(* Logix 5000 AddOnInstructionDefinition export AMP_Point_to_Point_IO; software revision 20.04 *)

TYPE AMP_Status_Word :   // Applied Motion Input Assembly Status Word
STRUCT
   Enabled : BOOL;   // Motor Enabled (Motor Disabled if this bit = 0)
   Sampling : BOOL;   // Sampling (for Quick Tuner)
   Drive_Fault : BOOL;   // Drive Fault (check Alarm Code)
   In_Position : BOOL;   // In Position (motor is in position)
   Moving : BOOL;   // Moving (motor is moving)
   Jogging : BOOL;   // Jogging (currently in jog mode)
   Stopping : BOOL;   // Stopping (in the process of stopping from a stop command)
   Waiting : BOOL;   // Waiting (for an input; executing a WI command)
   Saving : BOOL;   // Saving (parameter data is being saved)
   Alarm_Present : BOOL;   // Alarm present (check Alarm Code)
   Homing : BOOL;   // Homing (executing an SH command)
   Wait_Time : BOOL;   // Waiting (for time; executing a WD or WT command)
   Wizard_Running : BOOL;   // Wizard running (Timing Wizard is running)
   Checking_Encoder : BOOL;   // Checking encoder (Timing Wizard is running)
   Q_Program_Running : BOOL;   // Q Program is running
   Initializing : BOOL;   // Initializing (happens at power up) ; Servo Ready (for SV200 drives only)
END_STRUCT
END_TYPE

TYPE AMP_Input_Assembly_v2 :   // Applied Motion Drive Input Assembly Version 2.0
STRUCT
   Status_Code : DINT;   // Status Code
   Alarm_Code : DINT;   // Alarm Code
   Voltage : DINT;   // Supply Voltage (x0.1V)
   Current : DINT;   // Actual Current (mA)
   Temp : DINT;   // Drive Temperature (0.1 deg C)
   Encoder_Position : DINT;   // Encoder Position (20,000 counts = 1 shaft turn)
   Absolute_Position : DINT;   // Absolute Position (20,000 counts = 1 shaft turn)
   Position_Error : DINT;   // Position Error (counts)
   Actual_Velocity : DINT;   // Actual Velocity (rev/sec * 240, 0 when no encoder)
   Extended_Inputs : DINT;   // Input Status (Extended)
   Main_Board_Inputs : DINT;   // Input Status (Main board)
   Word11 : DINT;   // Reserved
   Analog_Input_1 : DINT;   // Analog Input 1 (ADC counts, 0=min V, 16383 = max V)
   Analog_Input_2 : DINT;   // Analog Input 2 (ADC counts, 0=min V, 16383 = max V)
END_STRUCT
END_TYPE

ADD_ON_INSTRUCTION AMP_Point_to_Point_IO   (* revision 1.0 *)
// Applied Motion - Point to Point Move with IO AOI
// Help:
// The Point-to-Point Move with I/O AOI executes moves involving up to 2 Input conditions and a possible output state change. The move variant can be any of the following:
// - FS - Feed to Sensor
// - FD - Feed to Double Sensor
// - FM - Feed to Sensor with Mask Distance
// - FY - Feed to Sensor with Safety Distance
// - FO - Feed to Length and Set Output
// - FE - Follow Encoder
// - SH - Seek Home
// All seven (7) of the above variants need exactly one I/O point except for FD which requires a second I/O point to be specified in the parameters.
VAR_IN_OUT
   Input : DINT[14]; {required}   // Drive Input Assembly
   Output : DINT[16]; {required}   // Drive Output Assembly
        [0]   // Command Word
        [1]   // Jog Speed (0.25 rev/min)
        [2]   // Jog Acceleration (10 rev/s/s)
        [3]   // Jog Deceleration (10 rev/s/s)
        [4]   // Point-to-Point Velocity (0.25 rev/min)
        [5]   // Point-to-Point Acceleration (10 rev/s/s)
        [6]   // Point-to-Point Deceleration (10 rev/s/s)
        [7]   // Point-to-Point Distance (Motor steps)
        [9]   // (2x ASCII Letters in 16 lower word)
        [10]   // Data/Register 1
        [11]   // Data/Register 2
END_VAR
VAR_INPUT
   RPI : DINT := 100; {visible}   // Drive Connection Request Packet Interval (milliseconds)
   Start : BOOL; {required}   // Start the Move
   Command : INT := 'FE'; {required}   // Command variant: FS/FD/FY/FM/FO/SH/FE
   IO1_Number : DINT; {required}   // Main Input/Output Number (0 = Encoder index, 1-8 = In/Out 1-8)
   IO1_Condition : SINT := 'R'; {required}   // Main Input/Output Condition/State H/L/R/F (High/Low/Rising Edge/Falling Edge)
   IO2_Number : DINT; {required}   // Second Input/Output Number (0 = Encoder index, 1-8 = In/Out 1-8)
   IO2_Condition : SINT; {required}   // Second Input/Output Condition/State H/L/R/F (High/Low/Rising Edge/Falling Edge)
   IO_Connector : DINT := 1; {required}   // I/O Connector (1=IN/OUT 1, 2=IN/OUT 2)
   Distance : DINT; {required}   // Distance to Move (negative = reverse)
   Speed : REAL; {required}   // Velocity of Move (rev/min)
   Acc : REAL; {required}   // Acceleration of Move (rev/s/s)
   Dec : REAL; {required}   // Deceleration (rev/s/s)
   Change_Distance : DINT; {required}   // Change Distance (steps, FY/FM/FO only)
   Change_Speed : REAL; {required}   // Velocity Change (rev/s) (FD only)
END_VAR
VAR_OUTPUT
   Sent : BOOL; {access Read Only, visible}   // Move has been sent to drive
   In_Progress : BOOL; {access Read Only, visible}   // Move in progress
   Done : BOOL; {access Read Only, visible}   // Move completed without errors - desired position reached
   Error : BOOL; {access Read Only, visible}   // Move failed to complete - drive not ready or faulted
   State : DINT := 10; {access Read Only}   // Internal state of progress
END_VAR
VAR
   Loc_StatusCode : AMP_Status_Word;
   Loc_CommandOff_Timer : TIMER;   // Timer to make sure command value was 0 before sending a new command
   Loc_CommandOn_Timer : TIMER;   // Timer to make sure command value is set long enough to be sent to drive
   Loc_Input_Assembly : AMP_Input_Assembly_v2; {access None}
   Loc_Start_ONS : BOOL; {access None}
   Loc_ChangeSpeed_Required : BOOL; {access None}
   Loc_ChangeDistance_Required : BOOL; {access None}
   Loc_IO1_Condition_Encoded : INT; {access None}
   Loc_IO1_Number_Encoded : INT; {access None}
   Loc_IO2_Condition_Encoded : INT; {access None}
   Loc_IO2_Number_Encoded : INT; {access None}
END_VAR

ROUTINE Logic   (* ladder *)
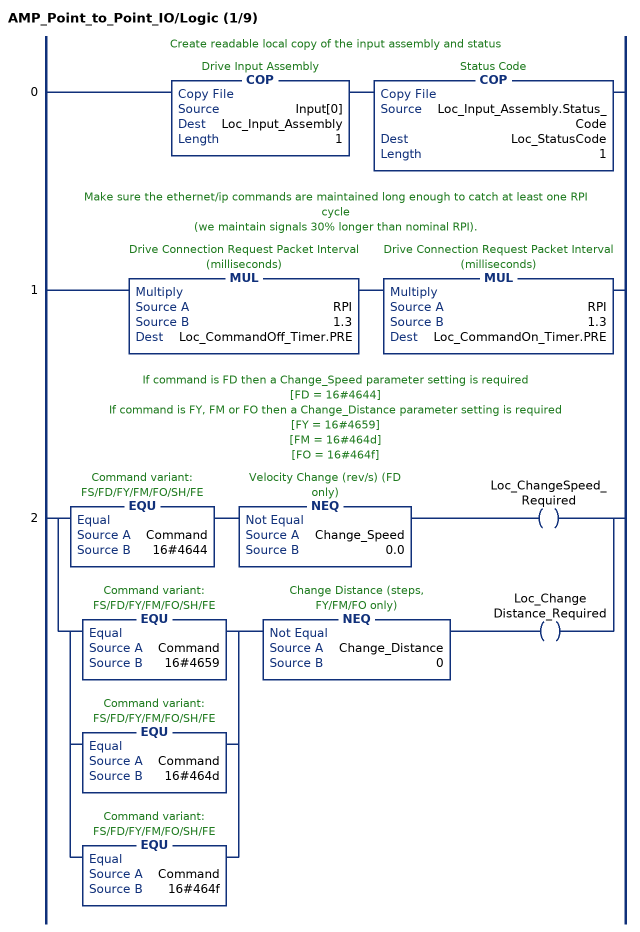
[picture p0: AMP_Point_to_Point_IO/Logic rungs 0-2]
   // Create readable local copy of the input assembly and status
   0: COP(Input[0],Loc_Input_Assembly,1)COP(Loc_Input_Assembly.Status_Code,Loc_StatusCode,1);
   // Make sure the ethernet/ip commands are maintained long enough to catch at least one RPI cycle
   // (we maintain signals 30% longer than nominal RPI).
   1: MUL(RPI,1.3,Loc_CommandOff_Timer.PRE)MUL(RPI,1.3,Loc_CommandOn_Timer.PRE);
   // If command is FD then a Change_Speed parameter setting is required
   // [FD = 16#4644]
   // If command is FY, FM or FO then a Change_Distance parameter setting is required
   // [FY = 16#4659]
   // [FM = 16#464d]
   // [FO = 16#464f]
   2: [EQU(Command,16#4644) NEQ(Change_Speed,0.0) OTE(Loc_ChangeSpeed_Required) ,[EQU(Command,16#4659) ,EQU(Command,16#464d) ,EQU(Command,16#464f) ] NEQ(Change_Distance,0) OTE(Loc_ChangeDistance_Required) ];
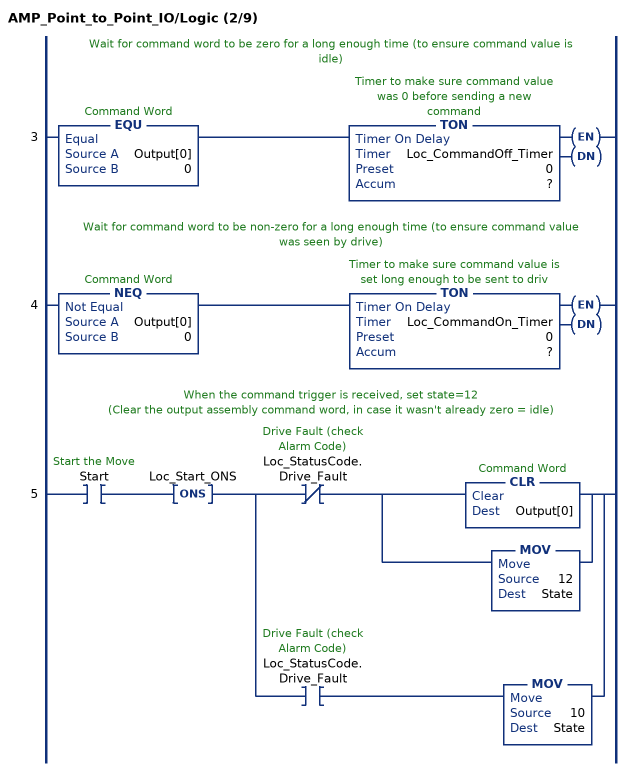
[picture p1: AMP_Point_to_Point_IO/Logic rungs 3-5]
   // Wait for command word to be zero for a long enough time (to ensure command value is idle)
   3: EQU(Output[0],0)TON(Loc_CommandOff_Timer,?,?);
   // Wait for command word to be non-zero for a long enough time (to ensure command value was seen by drive)
   4: NEQ(Output[0],0)TON(Loc_CommandOn_Timer,?,?);
   // When the command trigger is received, set state=12
   // (Clear the output assembly command word, in case it wasn't already zero = idle)
   5: XIC(Start)ONS(Loc_Start_ONS)[XIO(Loc_StatusCode.Drive_Fault) [CLR(Output[0]) ,MOV(12,State) ] ,XIC(Loc_StatusCode.Drive_Fault) MOV(10,State) ];
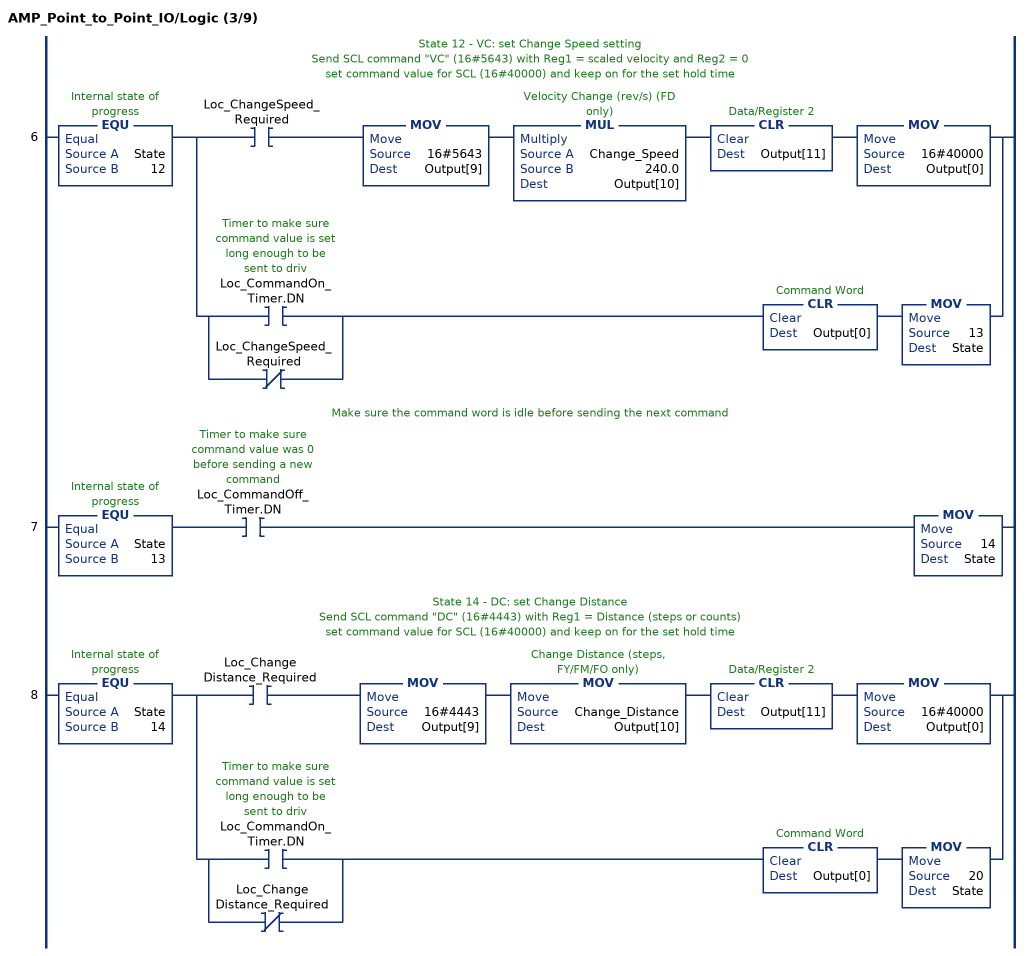
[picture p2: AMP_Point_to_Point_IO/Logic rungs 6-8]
   // State 12 - VC: set Change Speed setting
   // Send SCL command "VC" (16#5643) with Reg1 = scaled velocity and Reg2 = 0
   // set command value for SCL (16#40000) and keep on for the set hold time
   6: EQU(State,12)[XIC(Loc_ChangeSpeed_Required) MOV(16#5643,Output[9]) MUL(Change_Speed,240.0,Output[10]) CLR(Output[11]) MOV(16#40000,Output[0]) ,[XIC(Loc_CommandOn_Timer.DN) ,XIO(Loc_ChangeSpeed_Required) ] CLR(Output[0]) MOV(13,State) ];
   // Make sure the command word is idle before sending the next command
   7: EQU(State,13)XIC(Loc_CommandOff_Timer.DN)MOV(14,State);
   // State 14 - DC: set Change Distance
   // Send SCL command "DC" (16#4443) with Reg1 = Distance (steps or counts)
   // set command value for SCL (16#40000) and keep on for the set hold time
   8: EQU(State,14)[XIC(Loc_ChangeDistance_Required) MOV(16#4443,Output[9]) MOV(Change_Distance,Output[10]) CLR(Output[11]) MOV(16#40000,Output[0]) ,[XIC(Loc_CommandOn_Timer.DN) ,XIO(Loc_ChangeDistance_Required) ] CLR(Output[0]) MOV(20,State) ];
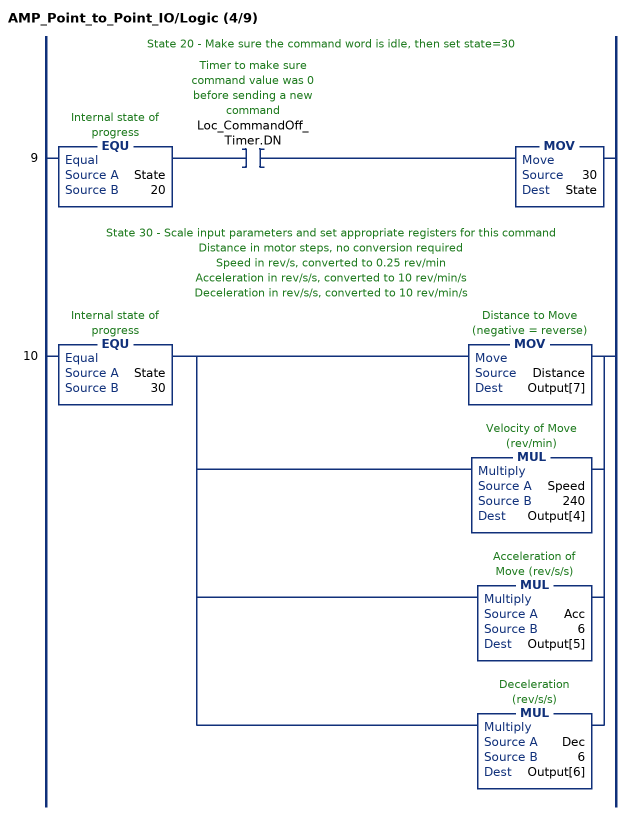
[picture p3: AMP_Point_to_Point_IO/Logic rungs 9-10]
   // State 20 - Make sure the command word is idle, then set state=30
   9: EQU(State,20)XIC(Loc_CommandOff_Timer.DN)MOV(30,State);
   // State 30 - Scale input parameters and set appropriate registers for this command
   // Distance in motor steps, no conversion required
   // Speed in rev/s, converted to 0.25 rev/min
   // Acceleration in rev/s/s, converted to 10 rev/min/s
   // Deceleration in rev/s/s, converted to 10 rev/min/s
   10: EQU(State,30)[MOV(Distance,Output[7]) ,MUL(Speed,240,Output[4]) ,MUL(Acc,6,Output[5]) ,MUL(Dec,6,Output[6]) ];
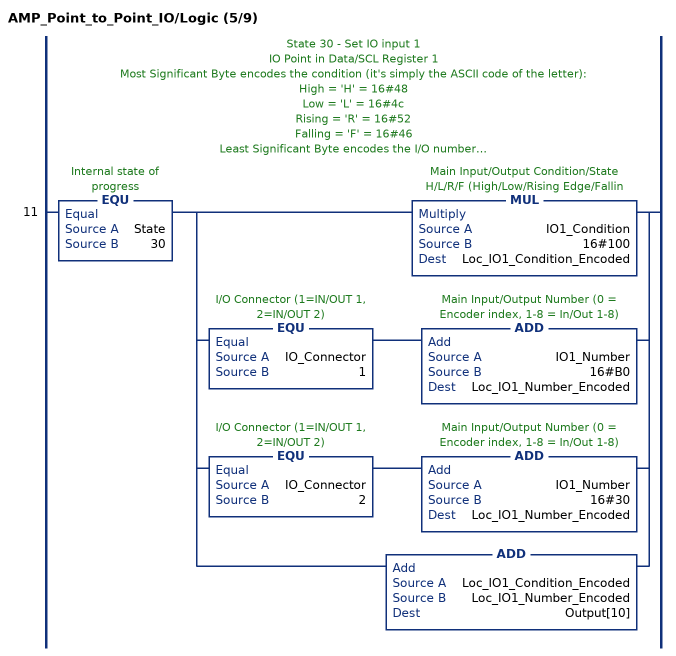
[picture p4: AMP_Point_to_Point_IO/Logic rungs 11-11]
   // State 30 - Set IO input 1
   // IO Point in Data/SCL Register 1
   // Most Significant Byte encodes the condition (it's simply the ASCII code of the letter):
   // High = 'H' = 16#48
   // Low = 'L' = 16#4c
   // Rising = 'R' = 16#52
   // Falling = 'F' = 16#46
   // Least Significant Byte encodes the I/O number:
   // 0xB0-0xBC for connector 1 (IN/OUT1) depending on provided I/O number 0-12 (0=encoder)
   // 0x30-0x3C for connector 2 (IN/OUT2) depending on provided I/O numbers 0-12 (0=encoder)
   11: EQU(State,30)[MUL(IO1_Condition,16#100,Loc_IO1_Condition_Encoded) ,EQU(IO_Connector,1) ADD(IO1_Number,16#B0,Loc_IO1_Number_Encoded) ,EQU(IO_Connector,2) ADD(IO1_Number,16#30,Loc_IO1_Number_Encoded) ,ADD(Loc_IO1_Condition_Encoded,Loc_IO1_Number_Encoded,Output[10]) ];
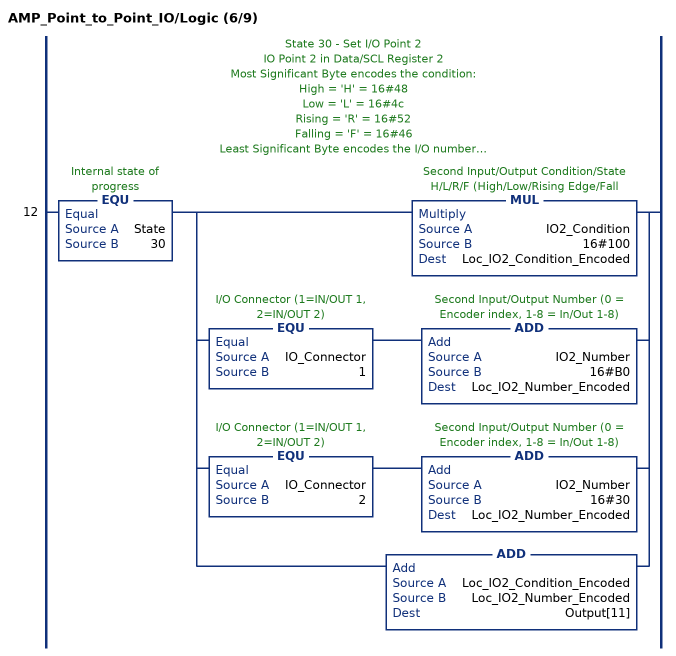
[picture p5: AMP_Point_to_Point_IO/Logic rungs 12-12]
   // State 30 - Set I/O Point 2
   // IO Point 2 in Data/SCL Register 2
   // Most Significant Byte encodes the condition:
   // High = 'H' = 16#48
   // Low = 'L' = 16#4c
   // Rising = 'R' = 16#52
   // Falling = 'F' = 16#46
   // Least Significant Byte encodes the I/O number:
   // 0xB0-0xBC for connector 1 (IN/OUT1) depending on provided I/O number 0-12 (0=encoder)
   // 0x30-0x3C for connector 2 (IN/OUT2) depending on provided I/O numbers 0-12 (0=encoder)
   12: EQU(State,30)[MUL(IO2_Condition,16#100,Loc_IO2_Condition_Encoded) ,EQU(IO_Connector,1) ADD(IO2_Number,16#B0,Loc_IO2_Number_Encoded) ,EQU(IO_Connector,2) ADD(IO2_Number,16#30,Loc_IO2_Number_Encoded) ,ADD(Loc_IO2_Condition_Encoded,Loc_IO2_Number_Encoded,Output[11]) ];
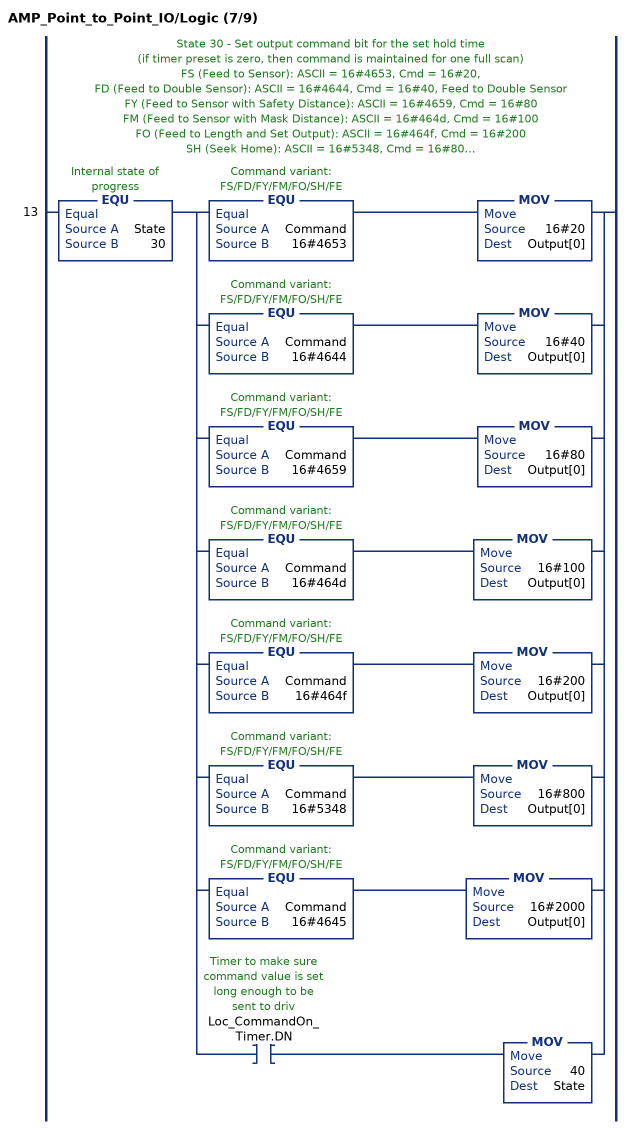
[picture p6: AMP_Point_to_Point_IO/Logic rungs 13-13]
   // State 30 - Set output command bit for the set hold time
   // (if timer preset is zero, then command is maintained for one full scan)
   // FS (Feed to Sensor): ASCII = 16#4653, Cmd = 16#20,
   // FD (Feed to Double Sensor): ASCII = 16#4644, Cmd = 16#40, Feed to Double Sensor
   // FY (Feed to Sensor with Safety Distance): ASCII = 16#4659, Cmd = 16#80
   // FM (Feed to Sensor with Mask Distance): ASCII = 16#464d, Cmd = 16#100
   // FO (Feed to Length and Set Output): ASCII = 16#464f, Cmd = 16#200
   // SH (Seek Home): ASCII = 16#5348, Cmd = 16#800
   // FE (Follow Encoder): ASCII = 16#4645, Cmd = 16#2000
   13: EQU(State,30)[[EQU(Command,16#4653) MOV(16#20,Output[0]) ,EQU(Command,16#4644) MOV(16#40,Output[0]) ,EQU(Command,16#4659) MOV(16#80,Output[0]) ,EQU(Command,16#464d) MOV(16#100,Output[0]) ,EQU(Command,16#464f) MOV(16#200,Output[0]) ,EQU(Command,16#5348) MOV(16#800,Output[0]) ,EQU(Command,16#4645) MOV(16#2000,Output[0]) ] ,XIC(Loc_CommandOn_Timer.DN) MOV(40,State) ];
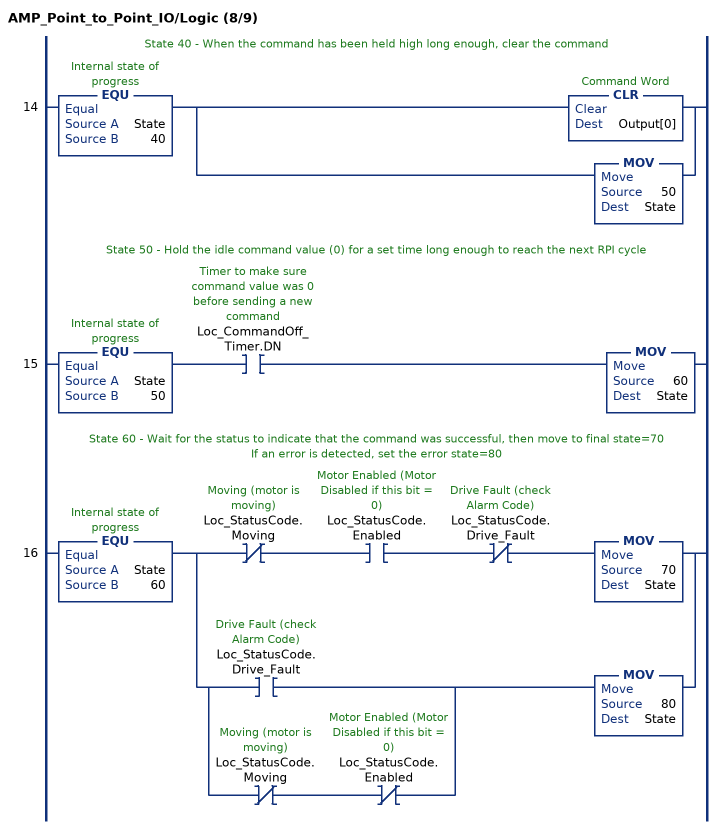
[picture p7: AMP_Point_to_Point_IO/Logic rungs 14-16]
   // State 40 - When the command has been held high long enough, clear the command
   14: EQU(State,40)[CLR(Output[0]) ,MOV(50,State) ];
   // State 50 - Hold the idle command value (0) for a set time long enough to reach the next RPI cycle
   15: EQU(State,50)XIC(Loc_CommandOff_Timer.DN)MOV(60,State);
   // State 60 - Wait for the status to indicate that the command was successful, then move to final state=70
   // If an error is detected, set the error state=80
   16: EQU(State,60)[XIO(Loc_StatusCode.Moving) XIC(Loc_StatusCode.Enabled) XIO(Loc_StatusCode.Drive_Fault) MOV(70,State) ,[XIC(Loc_StatusCode.Drive_Fault) ,XIO(Loc_StatusCode.Moving) XIO(Loc_StatusCode.Enabled) ] MOV(80,State) ];
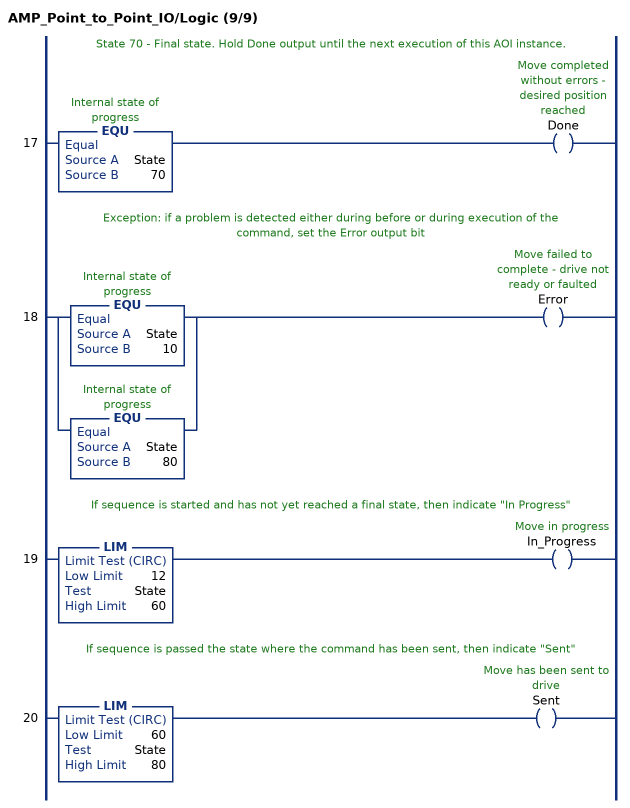
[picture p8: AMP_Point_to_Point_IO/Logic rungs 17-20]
   // State 70 - Final state. Hold Done output until the next execution of this AOI instance.
   17: EQU(State,70)OTE(Done);
   // Exception: if a problem is detected either during before or during execution of the command, set the Error output bit
   18: [EQU(State,10) ,EQU(State,80) ]OTE(Error);
   // If sequence is started and has not yet reached a final state, then indicate "In Progress"
   19: LIM(12,State,60)OTE(In_Progress);
   // If sequence is passed the state where the command has been sent, then indicate "Sent"
   20: LIM(60,State,80)OTE(Sent);
END_ROUTINE
END_ADD_ON_INSTRUCTION
